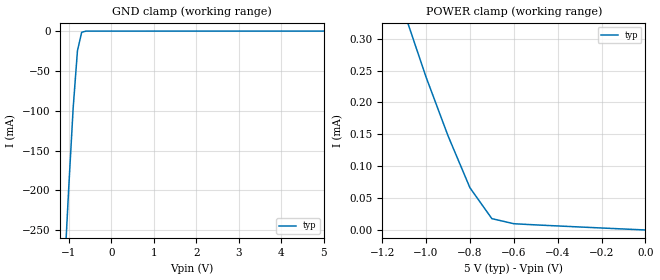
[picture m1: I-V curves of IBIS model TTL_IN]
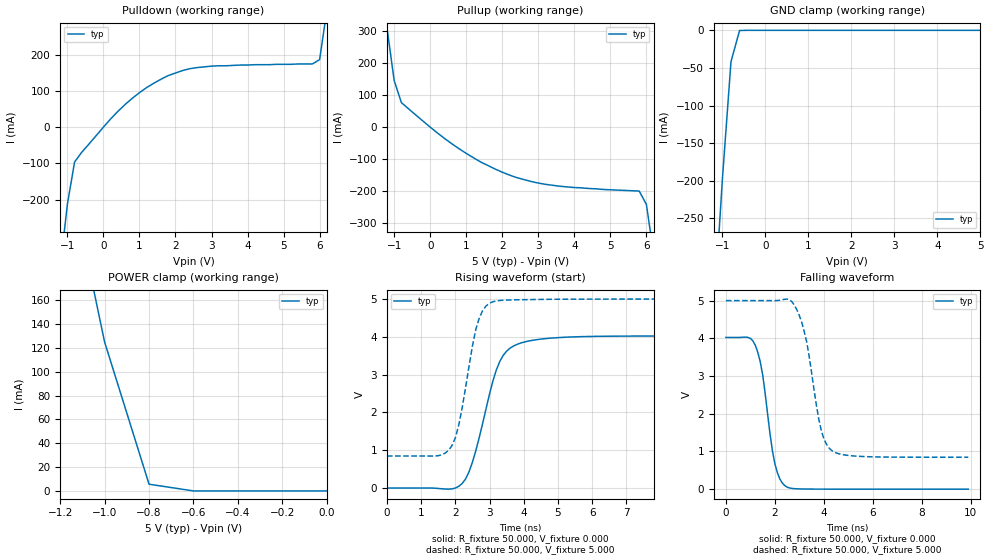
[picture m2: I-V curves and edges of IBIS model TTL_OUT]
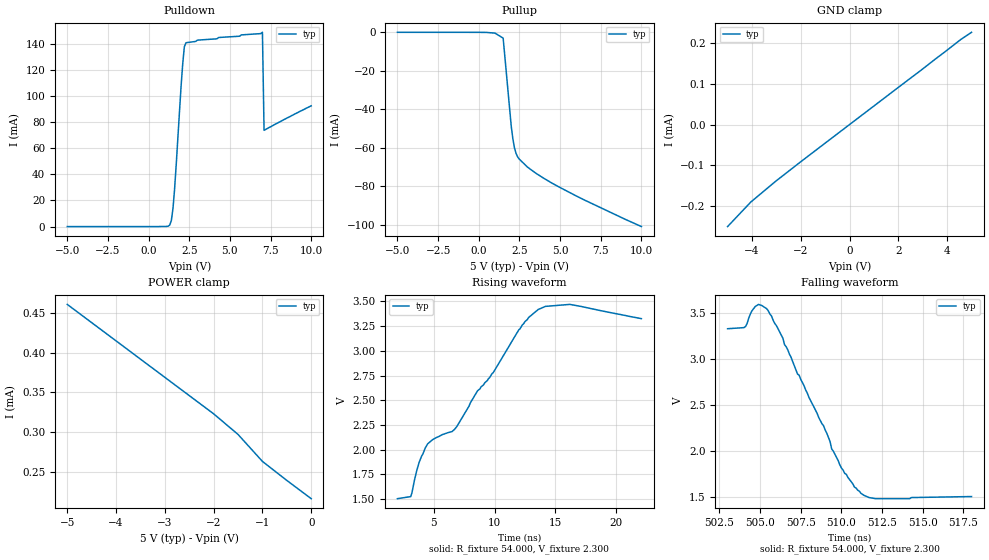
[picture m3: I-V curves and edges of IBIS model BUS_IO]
|   Texas Instruments Incorporated
|   Interface Products
|   IBIS Model for SN65LBC176A and SN75LBC176A
|   8D SOIC Package
[IBIS Ver]   3.2
[Comment char]   |_char
[File name]   lbc176ad.ibs
[File Rev]   1.0
[Date]   17Nov05
[Source]   File originated at Texas Instruments Incorporated.
   Interface Products Group.
[Notes]
[Disclaimer]
(C) Copyright Texas Instruments Incorporated 2005
   All rights reserved
  Texas Instruments Incorporated hereby grants the user of this IBIS
"model a non-exclusive, nontransferable license to use this IBIS model "
"under the following terms.  Before using this IBIS model, the user "
"should read this license.  If the user does not accept these terms, "
the IBIS model should be returned to Texas Instruments within 30 days.
  The user is granted this license only to use the IBIS model and
"is not granted rights to sell, load, rent, lease or license the IBIS"
"model in whole or in part, or in modified form to anyone other than"
user.  User may modify the IBIS model to suit its specific applications
but rights to derivative works and such modifications shall belong to
Texas Instruments.
"  This IBIS model is provided on an ""AS IS"" basis and Texas Instruments"
makes absolutely no warranty with respect to the information contained
"herein.  TEXAS INSTRUMENTS DISCLAIMS AND CUSTOMER WAIVES ALL WARRANTIES, "
"EXPRESS OR IMPLIED, INCLUDING WARRANTIES OF MERCHANTABILITY OR FITNESS "
FOR A PARTICULAR PURPOSE. The entire risk as to quality and performance
"is with the Customer. ACCORDINGLY, IN NO EVENT SHALL THE COMPANY BE LIABLE"
"FOR ANY DAMAGES, WHETHER IN CONTRACT OR TORT,INCLUDING ANY LOST PROFITS "
"OR OTHER INCIDENTAL, CONSEQUENTIAL, EXEMPLARY, OR PUNITIVE DAMAGES ARISING"
OUT OF THE USE OR APPLICATION OF THE IBIS model provided in this package.
"Further, Texas Instruments reserves the right to discontinue or make changes"
"without notice to any product herein to improve reliability, function, or "
design. Texas Instruments does not convey any license under patent rights
"or any other intellectual property rights, including those of third parties."
Contact Texas Instruments at ATTN:INTERFACE
[Copyright]   Copyright 2005, Texas Instruments, All Rights Reserved
[Component]   SN65LBC176AD
[Manufacturer]  Texas Instruments Incorporated
[Package]
|   typ   min   max
R_pkg   0.0   NA   NA
L_pkg   1.1nH   NA   NA
C_pkg   0.25pF   NA   NA
[Pin]   signal_name model_name   R_pin  L_pin  C_pin
1   R   TTL_OUT   0.093  1.53n  0.089p
2   RE/   TTL_IN   0.089  1.47n  0.084p
3   DE   TTL_IN   0.089  1.47n  0.084p
4   D   TTL_IN   0.093  1.53n  0.089p
5   GND   GND   0.044  0.94n  0.178p
6   A   BUS_IO   0.089  1.47n  0.084p
7   B   BUS_IO   0.089  1.47n  0.084p
8   VCC   POWER   0.044  0.94n  0.178p
[Diff_pin]   inv_pin   vdiff   tdelay_typ   tdelay_min   tdelay_max
| The 'xY' pin is Diff_pin and the 'xZ' pin is the inv_pin
6   7   NA   0 0 0
| Models and submodels in the file (3): TTL_IN (Input), TTL_OUT (Output), BUS_IO (I/O)
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|   TTL Input Model
[Model]   TTL_IN
Model_type   Input
|Signals   RE/, DE, D
Vinh = 2.0
Vinl = 0.8
|   typ   min   max
C_comp   17.0pF   NA   NA
|   typ   min   max
[Temperature Range]   25.0   NA   NA
[Voltage range]   5.0V   4.75V   5.25V
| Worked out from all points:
|   GND clamp passes 1 mA (typ) near -0.67 V on its own axis
[GND_clamp]
|   Voltage   I(typ)   I(min)   I(max)
-5V       -4.21A     NA         NA
-2V       -1.22A     NA         NA
-1V       -192mA     NA         NA
-900mV    -96.1mA    NA         NA
-800mV    -24.8mA    NA         NA
-700mV    -1.47mA    NA         NA
-500mV    -28.2uA    NA         NA
5V        11.6pA     NA         NA
[Power_clamp]
| Note that the[POWER_clamp]voltage table is referenced to Vcc
| and is calculated using Vtable=Vcc - Vmeasured.
|   Voltage   I(typ)   I(min)   I(max)
-5V       4.42mA     NA         NA
-2V       1.26mA     NA         NA
-1V       240uA      NA         NA
-900mV    148uA      NA         NA
-800mV    66.3uA     NA         NA
-700mV    17.8uA     NA         NA
-600mV    9.8uA      NA         NA
0V        11.6pA     NA         NA
|   TTL Input/Output  Model
[Model]   TTL_OUT
Model_type   Output
| Signals   R
Vmeas = 0V   |Reference voltage for timing measurements
Cref = 15pF   |Timing specification test load capacitance value
Rref = 1M   |Note: 1 M-Ohm load; single ended configuration
| variable   typ   min   max
C_comp   16.5pF   NA   NA
|   typ   min   max
[Temperature Range]   25.0   NA   NA
[Voltage range]   5.0V   4.75V   5.25V
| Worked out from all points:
|   slope of the pulldown table from 0 to 0.75 V, typ, clamps not added: 9.99 ohm
|   slope of the pullup table from 0 to 0.75 V, typ, clamps not added: 11.8 ohm
|   GND clamp passes 1 mA (typ) near -0.60 V on its own axis
|   POWER clamp passes 1 mA (typ) near -0.64 V on its own axis
|   rising waveform, R_fixture 50.000, V_fixture 0.000: 20-80 % time 703ps typ, NA min, NA max; typ from 0 V to 4.02 V
|   falling waveform, R_fixture 50.000, V_fixture 0.000: 20-80 % time 514ps typ, NA min, NA max; typ from 4.02 V to 0 V
|   rising waveform, R_fixture 50.000, V_fixture 5.000: 20-80 % time 490ps typ, NA min, NA max; typ from 0.847 V to 5 V
|   falling waveform, R_fixture 50.000, V_fixture 5.000: 20-80 % time 653ps typ, NA min, NA max; typ from 5 V to 0.847 V
[Pulldown]
|Voltage I(typ)   I(min)   I(max)
-5V       -4.117A    NA         NA
-1.2V     -388mA     NA         NA
-1V       -213mA     NA         NA
-800mV    -96.1mA    NA         NA
600mV     62.1mA     NA         NA
1.2V      109mA      NA         NA
1.8V      142mA      NA         NA
3V        168mA      NA         NA
5.8V      174mA      NA         NA
6V        186mA      NA         NA
6.2V      321mA      NA         NA
10V       4.037A     NA         NA
[Pullup]
|Voltage I(typ)   I(min)   I(max)
| Note that the[Pullup]voltage table is referenced to Vcc
| and is calculated using Vtable=Vcc - Vmeasured.
-5V       4.036A     NA         NA
-1.2V     311mA      NA         NA
-1V       146mA      NA         NA
-800mV    76.8mA     NA         NA
800mV     -67.5mA    NA         NA
1.4V      -109mA     NA         NA
2.2V      -150mA     NA         NA
3.6V      -185mA     NA         NA
5.8V      -200mA     NA         NA
6V        -242mA     NA         NA
6.2V      -398mA     NA         NA
10V       -4.117A    NA         NA
[GND_clamp]
|Voltage I(typ)   I(min)   I(max)
| Outputs in Tri-state.
-5V       -4.116A    NA         NA
-1.2V     -380mA     NA         NA
-1V       -198mA     NA         NA
-800mV    -41.7mA    NA         NA
-600mV    -211uA     NA         NA
5V        86.6pA     NA         NA
[POWER_clamp]
|Voltage I(typ)   I(min)   I(max)
| Note that the [POWER_clamp] voltage table is referenced to Vcc
| and is calculated using Vtable = Vcc - Vmeasured.
| Outputs in Tri-state.
-5V       4.035A     NA         NA
-1.2V     303mA      NA         NA
-1V       125mA      NA         NA
-800mV    5.64mA     NA         NA
-600mV    3.21uA     NA         NA
0V        86.6pA     NA         NA
[Ramp]
|   typ   min   max
dV/dt_r   4.0/1.220ns   NA   NA
dV/dt_f   4.0/1.248ns   NA   NA
R_load = 1MOhm   | note: Represents an open
[Rising Waveform]
R_fixture = 50.000
V_fixture = 0.000
C_fixture = 0.000
L_fixture = 0.000
|  time   V(typ)   V(min)   V(max)
0s        5.611nV    NA         NA
1.8ns     -30.02mV   NA         NA
2.2ns     119.9mV    NA         NA
2.4ns     427.7mV    NA         NA
2.5ns     684.7mV    NA         NA
3.2ns     3.126V     NA         NA
3.4ns     3.51V      NA         NA
3.8ns     3.799V     NA         NA
5.3ns     3.994V     NA         NA
9.9ns     4.023V     NA         NA
[Falling Waveform]
R_fixture = 50.000
V_fixture = 0.000
C_fixture = 0.000
L_fixture = 0.000
|  time   V(typ)   V(min)   V(max)
0s        4.023V     NA         NA
900ps     4.024V     NA         NA
1.2ns     3.817V     NA         NA
1.4ns     3.387V     NA         NA
1.5ns     3.038V     NA         NA
1.8ns     1.473V     NA         NA
2ns       675.1mV    NA         NA
2.2ns     275.2mV    NA         NA
2.5ns     54.57mV    NA         NA
9.9ns     5.611nV    NA         NA
[Rising Waveform]
R_fixture = 50.000
V_fixture = 5.000
C_fixture = 0.000
L_fixture = 0.000
|  time   V(typ)   V(min)   V(max)
0s        847.2mV    NA         NA
1.5ns     856mV      NA         NA
1.7ns     922.9mV    NA         NA
1.9ns     1.12V      NA         NA
2.1ns     1.665V     NA         NA
2.6ns     4.201V     NA         NA
2.8ns     4.696V     NA         NA
3ns       4.89V      NA         NA
3.8ns     4.981V     NA         NA
9.9ns     5V         NA         NA
[Falling Waveform]
R_fixture = 50.000
V_fixture = 5.000
C_fixture = 0.000
L_fixture = 0.000
|  time   V(typ)   V(min)   V(max)
0s        5V         NA         NA
2.7ns     4.967V     NA         NA
3ns       4.603V     NA         NA
3.3ns     3.902V     NA         NA
3.7ns     2.207V     NA         NA
3.9ns     1.547V     NA         NA
4.1ns     1.2V       NA         NA
4.4ns     990.8mV    NA         NA
5.7ns     862.9mV    NA         NA
9.9ns     847.2mV    NA         NA
[Model]   BUS_IO
Model_type   I/O
| Signals   A,B
Vinh = 0.2   |Positive going differential input voltage
Vinl = -0.2   |Negative going differential input voltage
Vmeas = 2.3V  |Reference voltage for timing measurements
Cref = 50pF   |Timing specification test load capacitance value
Rref = 54   |Note: 54 Ohm load; single ended configuration
|   typ   min   max
C_comp   18.5pF   NA   NA
|   typ   min   max
[Temperature Range]   25.0   NA   NA
[Voltage range]   5.0V   4.75V   5.25V
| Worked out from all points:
|   slope of the pulldown table from 0 to 0.75 V, typ, clamps not added: 18.8 kohm
|   slope of the pullup table from 0 to 0.75 V, typ, clamps not added: 3.08 kohm
|   rising waveform, R_fixture 54.000, V_fixture 2.300: 20-80 % time 7ns typ, NA min, NA max; typ from 1.5 V to 3.33 V
|   falling waveform, R_fixture 54.000, V_fixture 2.300: 20-80 % time 2.84ns typ, NA min, NA max; typ from 3.33 V to 1.5 V
[Power_clamp]
| Note that the[POWER_clamp]voltage table is referenced to Vcc
| and is calculated using Vtable=Vcc - Vmeasured.
|   Voltage   I(typ)   I(min)   I(max)
-5V       461uA      NA         NA
-4.5V     438uA      NA         NA
-4V       415uA      NA         NA
-3.5V     392uA      NA         NA
-3V       369uA      NA         NA
-2.5V     346uA      NA         NA
-2V       323uA      NA         NA
-1.5V     297uA      NA         NA
-1V       263uA      NA         NA
-500mV    239uA      NA         NA
0V        216uA      NA         NA
[GND_clamp]
|   Voltage   I(typ)   I(min)   I(max)
-5V       -250uA     NA         NA
-4.05V    -190uA     NA         NA
-3.05V    -140uA     NA         NA
4.55V     208uA      NA         NA
5V        226uA      NA         NA
[Pulldown]
|   Voltage   I(typ)   I(min)   I(max)
-5V       -560pA     NA         NA
1.3V      1.13mA     NA         NA
1.4V      4.65mA     NA         NA
1.5V      13.9mA     NA         NA
1.6V      29mA       NA         NA
2V        108mA      NA         NA
2.1V      125mA      NA         NA
2.2V      138mA      NA         NA
2.3V      141mA      NA         NA
7V        149mA      NA         NA
7.1V      73.8mA     NA         NA
10V       92.6mA     NA         NA
[Pullup]
|   Voltage   I(typ)   I(min)   I(max)
| Note that the[Pullup]voltage table is referenced to Vcc
| and is calculated using Vtable=Vcc - Vmeasured.
-5V       16.6uA     NA         NA
500mV     -60.3uA    NA         NA
1V        -426uA     NA         NA
1.5V      -3.01mA    NA         NA
2V        -49mA      NA         NA
2.1V      -55.5mA    NA         NA
2.2V      -60.2mA    NA         NA
2.4V      -64.9mA    NA         NA
3V        -70.1mA    NA         NA
4.5V      -78.4mA    NA         NA
6.5V      -87.2mA    NA         NA
10V       -101mA     NA         NA
[Ramp]
|   typ   min   max
dV/dt_r   1.77v/7ns   NA   NA
dV/dt_f   1.60v/3.2ns   NA   NA
R_load = 54ohm  | Note: The measurement is single-ended with respect
|   to ground.
[Rising Waveform]
R_fixture = 54.000
V_fixture = 2.300
C_fixture = 0.000
L_fixture = 0.000
|  time   V(typ)   V(min)   V(max)
2ns       1.505V     NA         NA
3.1ns     1.526V     NA         NA
3.8ns     1.876V     NA         NA
4.5ns     2.061V     NA         NA
6.7ns     2.205V     NA         NA
9.9ns     2.781V     NA         NA
12ns      3.213V     NA         NA
13.6ns    3.419V     NA         NA
16.2ns    3.47V      NA         NA
22.1ns    3.326V     NA         NA
[Falling Waveform]
R_fixture = 54.000
V_fixture = 2.300
C_fixture = 0.000
L_fixture = 0.000
|  time   V(typ)   V(min)   V(max)
503ns     3.326V     NA         NA
504.1ns   3.349V     NA         NA
504.5ns   3.521V     NA         NA
504.9ns   3.59V      NA         NA
505.4ns   3.544V     NA         NA
508.9ns   2.273V     NA         NA
509.4ns   2.021V     NA         NA
511.2ns   1.54V      NA         NA
512.1ns   1.482V     NA         NA
518ns     1.505V     NA         NA
